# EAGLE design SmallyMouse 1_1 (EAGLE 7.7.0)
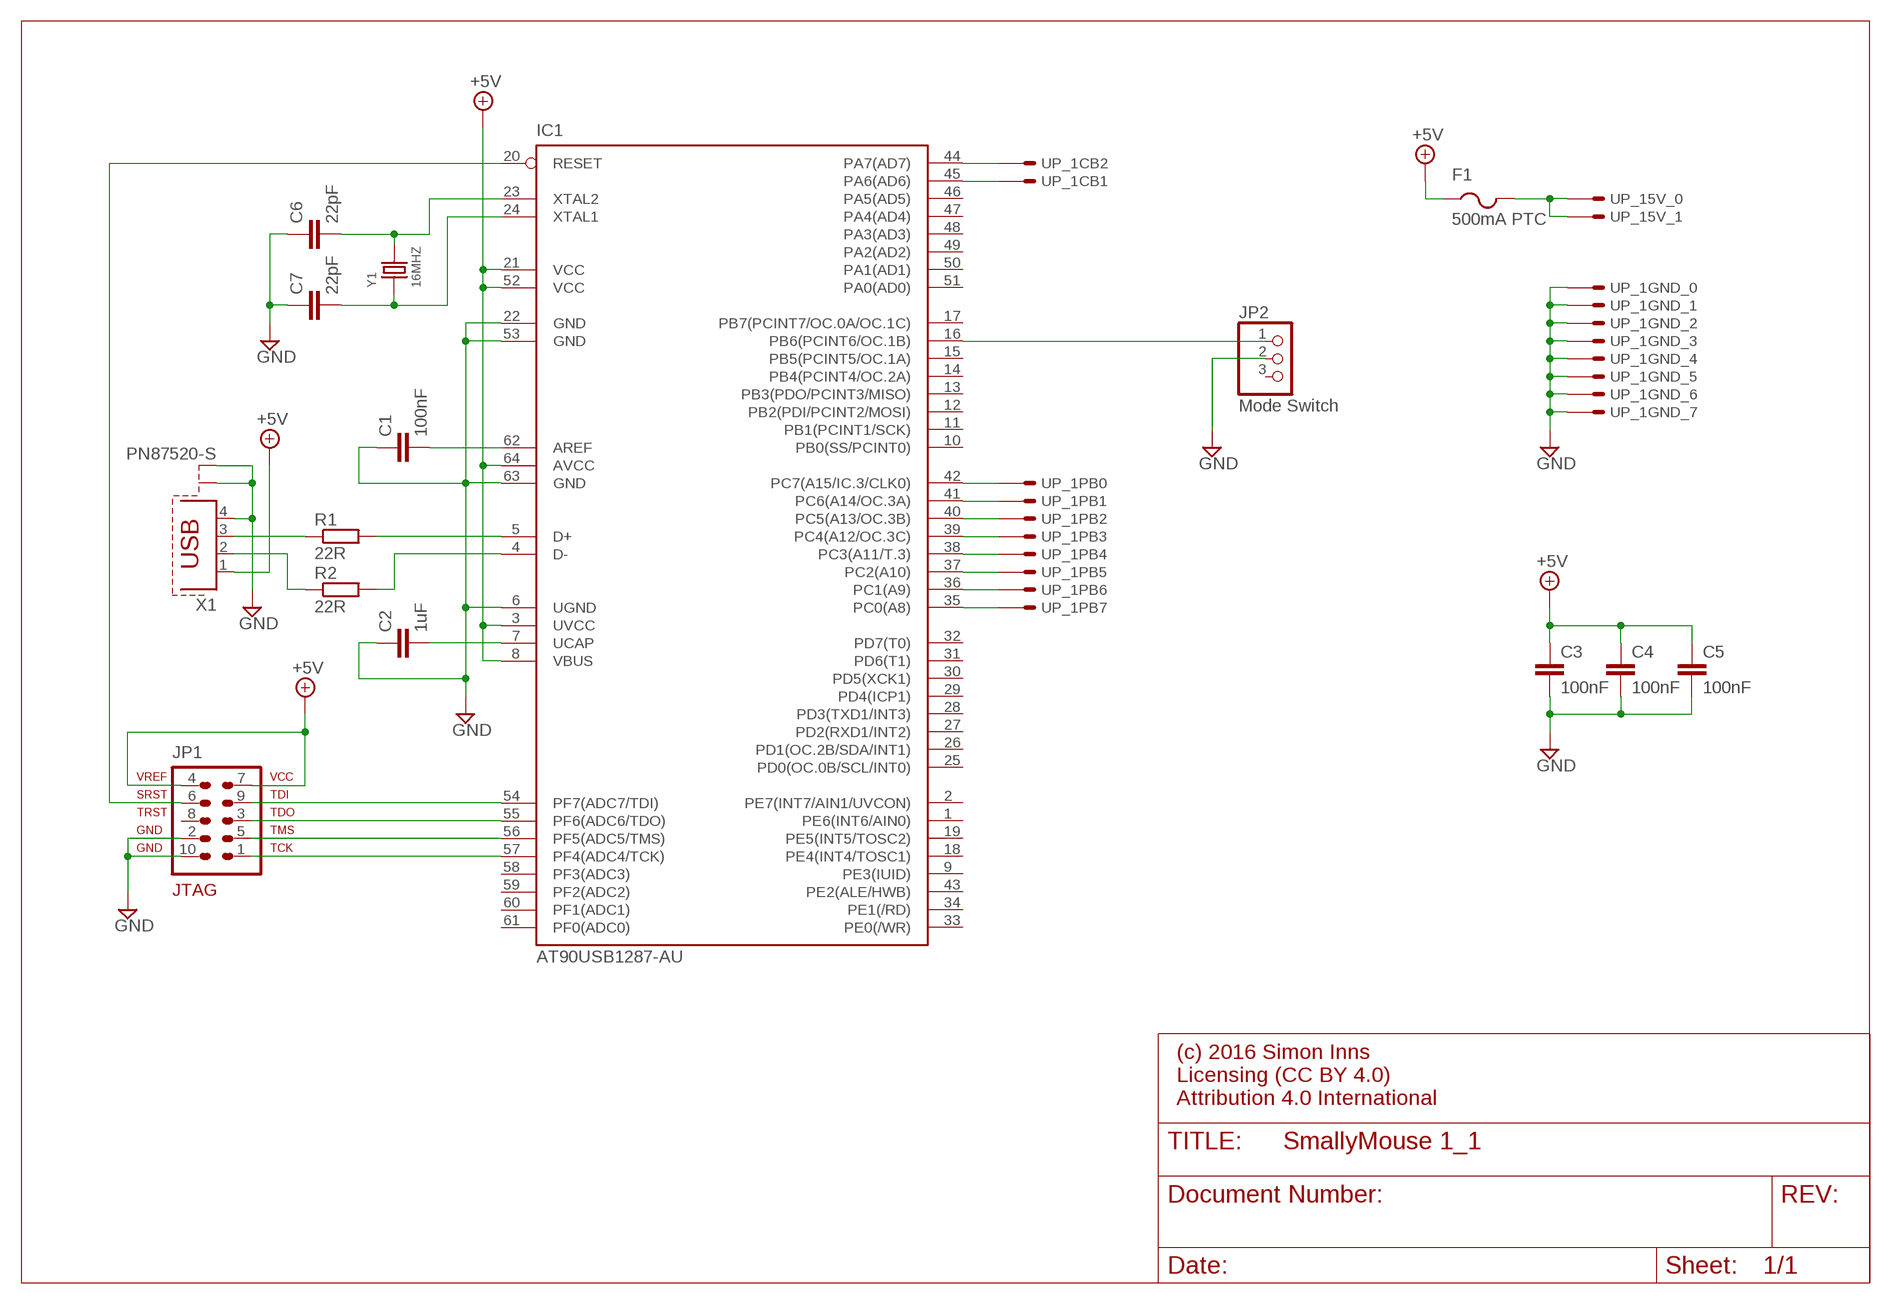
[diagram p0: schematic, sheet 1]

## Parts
C1  100nF  C-EUC0805  [C0805]
C2  1uF  C-EUC0805  [C0805]
C3  100nF  C-EUC0805  [C0805]
C4  100nF  C-EUC0805  [C0805]
C5  100nF  C-EUC0805  [C0805]
C6  22pF  C-EUC0805  [C0805]
C7  22pF  C-EUC0805  [C0805]
F1  500mA PTC  PTCFUSE-1812  [1812]
IC1  AT90USB1287-AU  [TQFP64]
JP1  AVR-JTAG-10  [AVR-JTAG-10]
JP2  Mode Switch  PINHD-1X3/90  [1X03/90]
R1  22R  R-EU_M1206  [M1206]
R2  22R  R-EU_M1206  [M1206]
UP_1  BBC_USERPORT  [20_PIN_HEADER]
X1  PN87520-S  [PN87520-S]
Y1  16MHZ  SMD-CRYSTAL-16MHZ-8PF-20PPM-40R(2P-5.0X3.2MM)  [X2-SMD-5.0X3.2X1.3MM]

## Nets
+5V: C3.1 C4.1 C5.1 F1.1 IC1.3(UVCC) IC1.8(VBUS) IC1.21(VCC) IC1.52(VCC) IC1.64(AVCC) JP1.4 JP1.7 X1.1
GND: C1.1 C2.1 C3.2 C4.2 C5.2 C6.1 C7.1 IC1.6(UGND) IC1.22(GND) IC1.53(GND) IC1.63(GND) JP1.2 JP1.10 JP2.2 UP_1.5 UP_1.7 UP_1.9 UP_1.11 UP_1.13 UP_1.15 UP_1.17 UP_1.19 X1.4 X1.S1 X1.S2
N$1: IC1.42(PC7(A15/IC.3/CLK0)) UP_1.6
N$2: IC1.41(PC6(A14/OC.3A)) UP_1.8
N$3: IC1.40(PC5(A13/OC.3B)) UP_1.10
N$4: IC1.39(PC4(A12/OC.3C)) UP_1.12
N$5: IC1.38(PC3(A11/T.3)) UP_1.14
N$6: IC1.37(PC2(A10)) UP_1.16
N$7: IC1.36(PC1(A9)) UP_1.18
N$8: IC1.35(PC0(A8)) UP_1.20
N$9: IC1.44(PA7(AD7)) UP_1.4
N$10: IC1.45(PA6(AD6)) UP_1.2
N$11: IC1.54(PF7(ADC7/TDI)) JP1.9
N$12: IC1.55(PF6(ADC6/TDO)) JP1.3
N$13: IC1.56(PF5(ADC5/TMS)) JP1.5
N$14: IC1.57(PF4(ADC4/TCK)) JP1.1
N$15: IC1.5(D+) R1.2
N$16: IC1.4(D-) R2.2
N$17: IC1.20(RESET) JP1.6
N$18: IC1.16(PB6(PCINT6/OC.1B)) JP2.1
N$19: F1.2 UP_1.1 UP_1.3
N$26: R1.1 X1.3
N$27: R2.1 X1.2
N$29: C1.2 IC1.62(AREF)
N$31: C2.2 IC1.7(UCAP)
N$32: C6.2 IC1.23(XTAL2) Y1.2
N$33: C7.2 IC1.24(XTAL1) Y1.1
Unconnected: IC1.1(PE6(INT6/AIN0)) IC1.2(PE7(INT7/AIN1/UVCON)) IC1.9(PE3(IUID)) IC1.10(PB0(SS/PCINT0)) IC1.11(PB1(PCINT1/SCK)) IC1.12(PB2(PDI/PCINT2/MOSI)) IC1.13(PB3(PDO/PCINT3/MISO)) IC1.14(PB4(PCINT4/OC.2A)) IC1.15(PB5(PCINT5/OC.1A)) IC1.17(PB7(PCINT7/OC.0A/OC.1C)) IC1.18(PE4(INT4/TOSC1)) IC1.19(PE5(INT5/TOSC2)) IC1.25(PD0(OC.0B/SCL/INT0)) IC1.26(PD1(OC.2B/SDA/INT1)) IC1.27(PD2(RXD1/INT2)) IC1.28(PD3(TXD1/INT3)) IC1.29(PD4(ICP1)) IC1.30(PD5(XCK1)) IC1.31(PD6(T1)) IC1.32(PD7(T0)) IC1.33(PE0(/WR)) IC1.34(PE1(/RD)) IC1.43(PE2(ALE/HWB)) IC1.46(PA5(AD5)) IC1.47(PA4(AD4)) IC1.48(PA3(AD3)) IC1.49(PA2(AD2)) IC1.50(PA1(AD1)) IC1.51(PA0(AD0)) IC1.58(PF3(ADC3)) IC1.59(PF2(ADC2)) IC1.60(PF1(ADC1)) IC1.61(PF0(ADC0)) JP1.8 JP2.3

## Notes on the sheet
- (c) 2016 Simon Inns
  Licensing (CC BY 4.0)
  Attribution 4.0 International

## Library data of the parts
C1-C7 = rcl:C-EU: CAPACITOR, European symbol
F1 = adafruit:PTCFUSE: PTC fuses, resettable thermistors
IC1 = at90usb:AT90USB1287-*: Atmel AT90USB1287 AVR Microcontroller with USB Interface and 128kB Flash Memory
JP1 = avr-7:AVR-JTAG-10: AVR JTAG Debug/Programming Header
JP2 = pinhead:PINHD-1X3: PIN HEADER
R1 R2 = rcl:R-EU_: RESISTOR, European symbol
UP_1 = BBC Micro:BBC_USERPORT: BBC Micro user port
X1 = con-berg:PN87520-S; OC_FARNELL: unknown; OC_NEWARK: unknown
Y1 = Seeed-OPL-Crystal-Oscillator:SMD-CRYSTAL-16MHZ-8PF-20PPM-40R(2P-5.0X3.2MM): 306010054; MPN: X053201602002

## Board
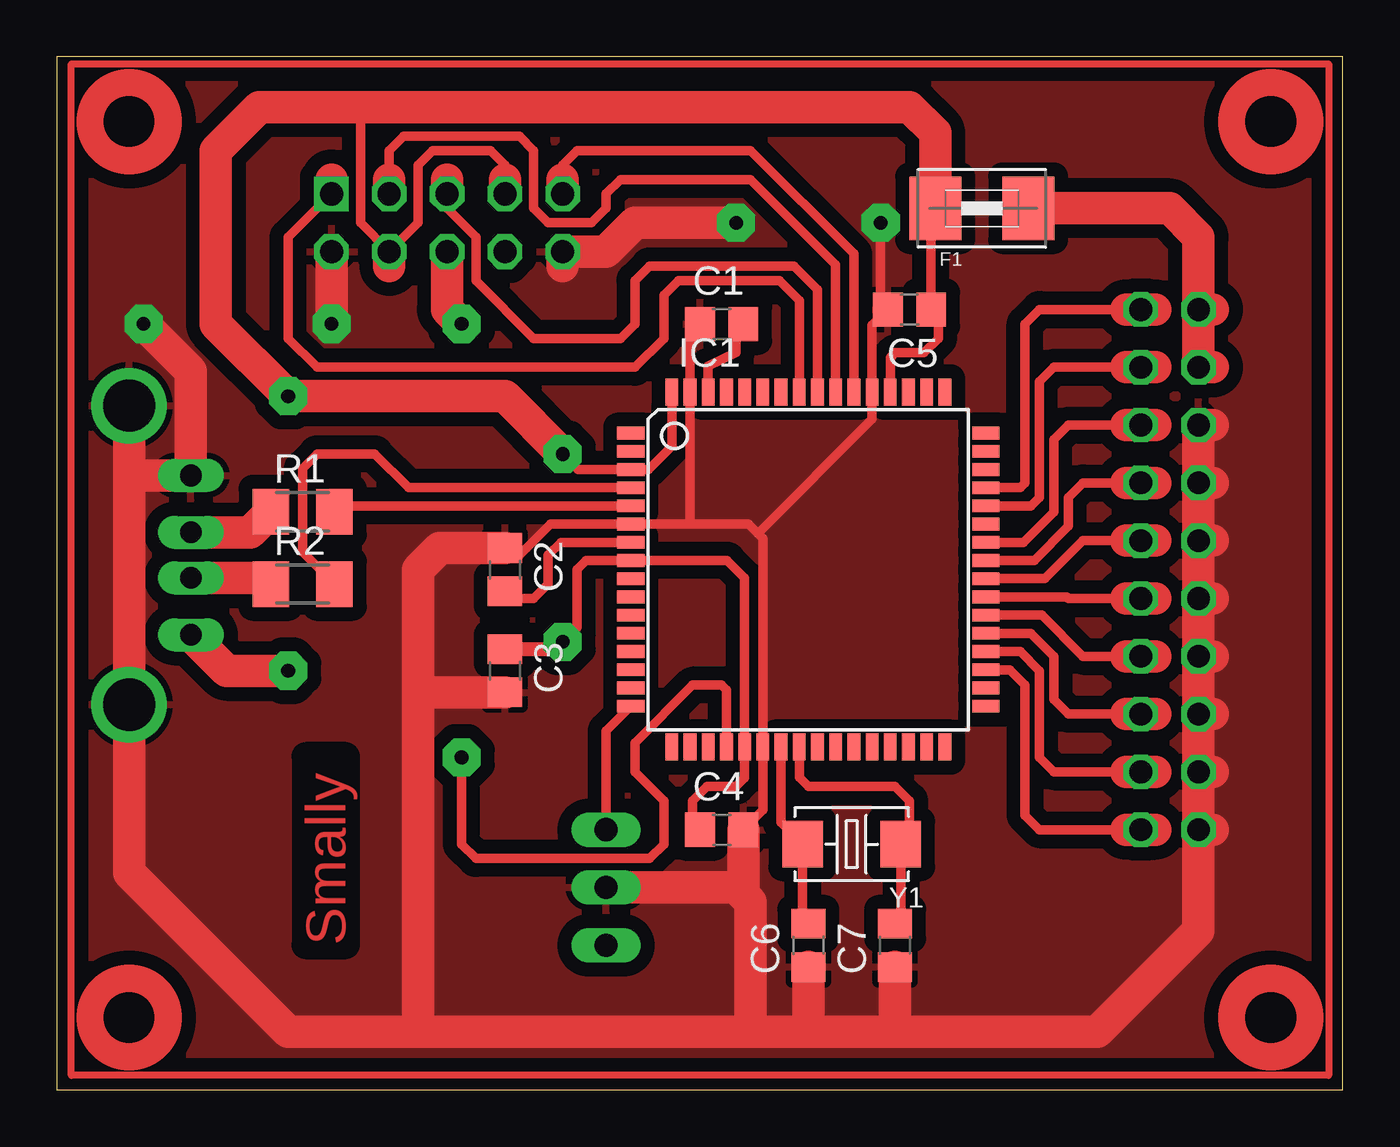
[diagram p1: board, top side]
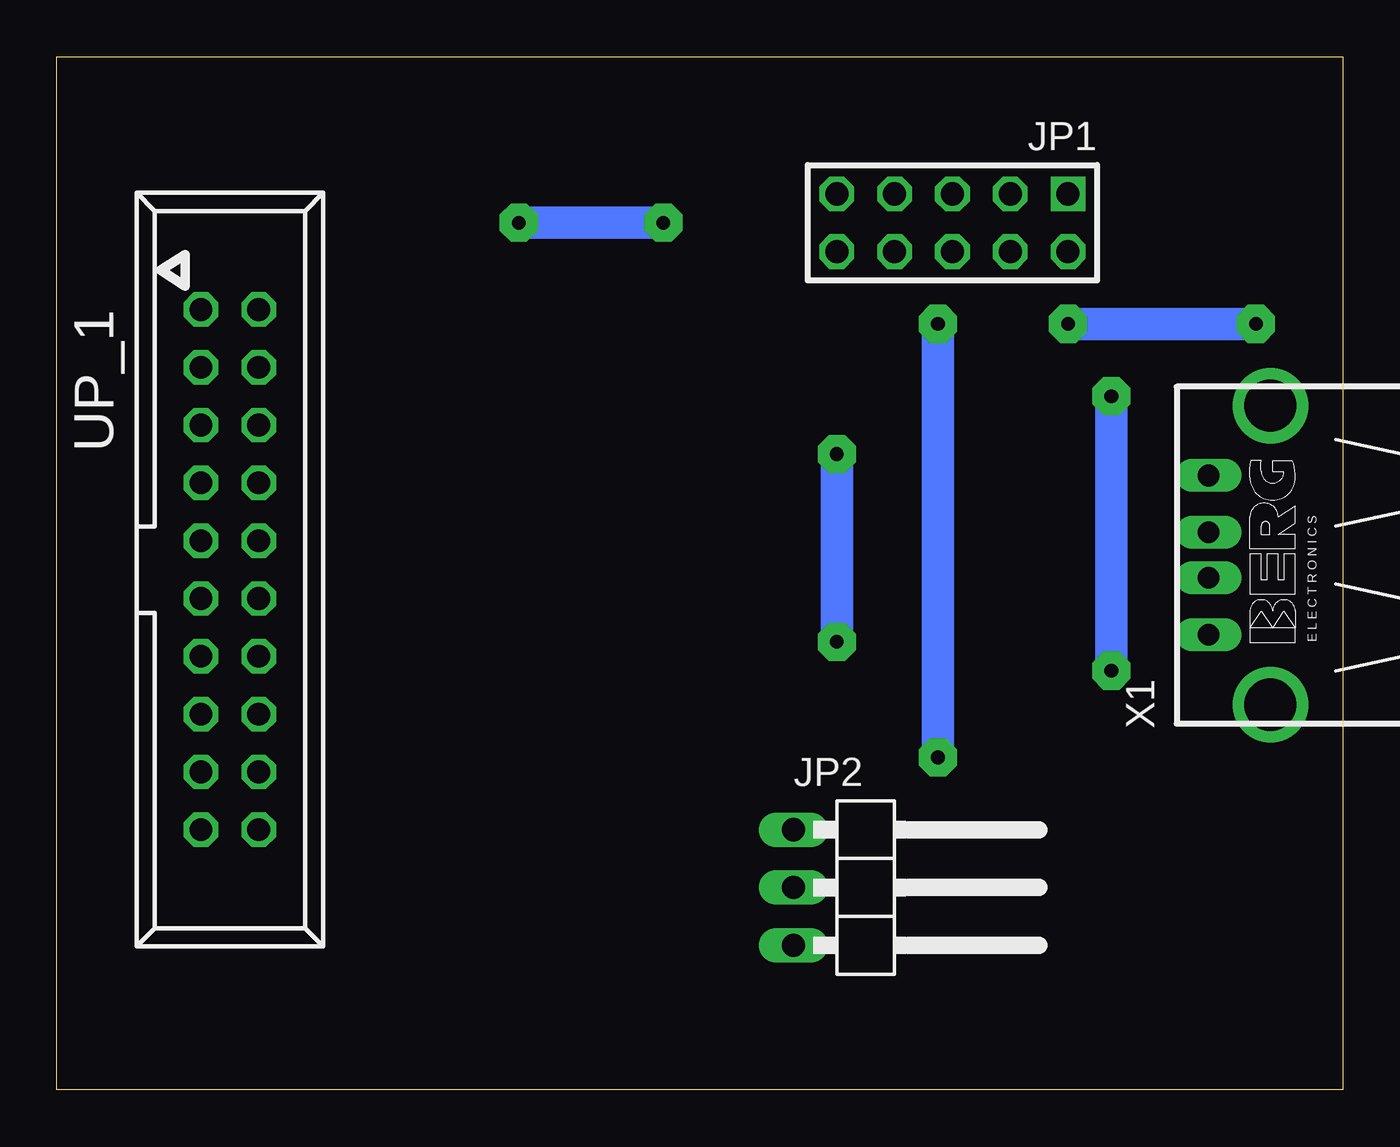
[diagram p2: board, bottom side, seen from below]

Size 56.49 x 45.39 mm. Coordinates in mm from the lower left corner, seen from the top.
Outline: 0,0 56.49,0 56.49,45.39 0,45.39 0,0
Copper layers (1*16): Top 0.035mm / dielectric 1.5mm / Bottom 0.035mm
Design rules "default": minimum track width 10mil, minimum drill 24mil, track to track 8mil, track to pad 8mil, pad to pad 8mil, via to via 8mil, smd to smd 8mil, copper to edge 40mil, drill to drill 8mil, minimum pad ring 10mil, minimum via ring 8mil, stop-mask expansion 4mil, vias tented up to drill 0mil, thermal gap 10mil
tRestrict: area 2.3,41.6 to 4.1,43.4; area 2.3,2.3 to 4.1,4.1; area 52.4,2.3 to 54.2,4.1; area 52.4,41.6 to 54.2,43.4

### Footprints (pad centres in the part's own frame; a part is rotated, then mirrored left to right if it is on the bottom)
C0805 = smd 1.3 x 1.5: 1 -0.95,0; 2 0.95,0
1812 = smd 2.286 x 2.794: 1 -2.046,0; 2 2.046,0
TQFP64 = smd 1.194 x 0.559: 1 -7.8,6; 2 -7.8,5.2; 3 -7.8,4.4; 4 -7.8,3.6; 5 -7.8,2.8; 6 -7.8,2; 7 -7.8,1.2; 8 -7.8,0.4; 9 -7.8,-0.4; 10 -7.8,-1.2; 11 -7.8,-2; 12 -7.8,-2.8; 13 -7.8,-3.6; 14 -7.8,-4.4; 15 -7.8,-5.2; 16 -7.8,-6; 33 7.8,-6; 34 7.8,-5.2; 35 7.8,-4.4; 36 7.8,-3.6; 37 7.8,-2.8; 38 7.8,-2; 39 7.8,-1.2; 40 7.8,-0.4; 41 7.8,0.4; 42 7.8,1.2; 43 7.8,2; 44 7.8,2.8; 45 7.8,3.6; 46 7.8,4.4; 47 7.8,5.2; 48 7.8,6 | smd 0.559 x 1.194: 17 -6,-7.8; 18 -5.2,-7.8; 19 -4.4,-7.8; 20 -3.6,-7.8; 21 -2.8,-7.8; 22 -2,-7.8; 23 -1.2,-7.8; 24 -0.4,-7.8; 25 0.4,-7.8; 26 1.2,-7.8; 27 2,-7.8; 28 2.8,-7.8; 29 3.6,-7.8; 30 4.4,-7.8; 31 5.2,-7.8; 32 6,-7.8; 49 6,7.8; 50 5.2,7.8; 51 4.4,7.8; 52 3.6,7.8; 53 2.8,7.8; 54 2,7.8; 55 1.2,7.8; 56 0.4,7.8; 57 -0.4,7.8; 58 -1.2,7.8; 59 -2,7.8; 60 -2.8,7.8; 61 -3.6,7.8; 62 -4.4,7.8; 63 -5.2,7.8; 64 -6,7.8
AVR-JTAG-10 = drill 1.016 square: 1 -5.08,-1.27 | drill 1.016 octagon: 2 -5.08,1.27; 3 -2.54,-1.27; 4 -2.54,1.27; 5 0,-1.27; 6 0,1.27; 7 2.54,-1.27; 8 2.54,1.27; 9 5.08,-1.27; 10 5.08,1.27
1X03/90 = drill 1.016 long: 1 -2.54,-3.81; 2 0,-3.81; 3 2.54,-3.81
M1206 = smd 1.6 x 2: 1 -1.4,0; 2 1.4,0
20_PIN_HEADER = drill 1 octagon: 1 -11.43,-1.27; 2 -11.43,1.27; 3 -8.89,-1.27; 4 -8.89,1.27; 5 -6.35,-1.27; 6 -6.35,1.27; 7 -3.81,-1.27; 8 -3.81,1.27; 9 -1.27,-1.27; 10 -1.27,1.27; 11 1.27,-1.27; 12 1.27,1.27; 13 3.81,-1.27; 14 3.81,1.27; 15 6.35,-1.27; 16 6.35,1.27; 17 8.89,-1.27; 18 8.89,1.27; 19 11.43,-1.27; 20 11.43,1.27
PN87520-S = drill 0.95 long: 1 -3.5,2.71; 2 -1,2.71; 3 1,2.71; 4 3.5,2.71 | drill 2.3 pad 2.9: S1 -6.57,0; S2 6.57,0
X2-SMD-5.0X3.2X1.3MM = smd 1.778 x 2.032: 1 -2.159,0; 2 2.159,0

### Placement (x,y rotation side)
C1  29.21,33.66 0 top
C2  19.68,22.86 270 top
C3  19.68,18.41 270 top
C4  29.21,11.43 0 top
C5  37.47,34.29 180 top
C6  33.02,6.35 90 top
C7  36.83,6.35 90 top
F1  40.64,38.73 0 top
IC1  33.02,22.86 0 top
JP1  17.14,38.1 180 bottom
JP2  20.32,8.89 270 bottom
R1  10.79,25.4 0 top
R2  10.79,22.23 0 top
UP_1  48.9,22.86 270 bottom
X1  3.17,23.5 90 bottom
Y1  34.92,10.79 180 top

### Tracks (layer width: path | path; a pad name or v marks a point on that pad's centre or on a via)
+5V  (via drill 0.6 pad 1.68)
  Top 0.406: C4.1 27.94,11.75 27.94,12.7 28.57,13.34 29.84,13.34 30.22,13.71 IC1.21 30.22,22.48 29.45,23.26 IC1.8 23.26,23.26 22.86,22.86 22.86,20.32 v22.23,19.68 | IC1.52 36.62,32.17 36.83,32.38 38.1,32.38 38.73,33.02 38.73,33.97 C5.1 38.41,38.56 F1.1 | IC1.64 27.02,28.29 25.99,27.26 IC1.3 22.91,27.26 v22.23,27.94 | 19.68,40.01 19.68,40.64 19.05,41.27 16.51,41.27 15.88,40.64 15.88,38.1 JP1.4 13.34,38.1 13.34,43.18
  Top 0.61: C3.1 21.91,19.36 v22.23,19.68
  Top 1.422: F1.1 38.59,42.05 37.47,43.18 13.34,43.18 8.89,43.18 6.99,41.27 6.99,33.66 v10.16,30.48 19.68,30.48 v22.23,27.94 | X1.1 7.46,18.41 v10.16,18.41 | JP1.7 19.68,40.01 | JP1.4 14.61,36.2
  Bottom 1.422: v10.16,18.41 v10.16,30.48 | v22.23,19.68 v22.23,27.94
GND  (via drill 0.6 pad 1.68)
  Top 0.406: C4.2 31.02,12.29 IC1.22 31.02,24.23 30.8,24.45 | C1.1 27.82,33.85 IC1.63 27.82,24.98 27.94,24.86 | 30.8,24.45 30.39,24.86 27.94,24.86 | 27.94,24.86 IC1.6 21.68,24.86 20.32,23.5 19.68,24.13 | 30.8,24.45 35.82,29.47 IC1.53 35.82,33.59 C5.2 36.2,34.61 v36.2,38.1
  Top 1.422: UP_1.19 UP_1.17 | UP_1.17 UP_1.15 | UP_1.15 UP_1.13 | UP_1.13 UP_1.11 | UP_1.11 UP_1.9 | UP_1.9 UP_1.7 | UP_1.7 UP_1.5 50.8,29.21 | 33.02,2.54 36.83,2.54 | 36.83,2.54 45.72,2.54 50.16,6.99 UP_1.19 | JP2.2 29.84,8.89 30.16,8.57 | 15.88,2.54 10.16,2.54 3.17,9.53 X1.S1 3.17,27 | 15.88,2.54 30.48,2.54 | 30.48,2.54 33.02,2.54 | 3.17,27 X1.S2 | 3.17,27 X1.4 5.88,31.58 v3.81,33.66 | C2.1 16.82,23.81 15.88,22.86 15.88,17.14 | 15.88,17.14 15.88,2.54 | C3.2 16.2,17.46 15.88,17.14 | C7.1 36.83,2.54 | C6.1 33.02,2.54 | 30.48,2.54 30.48,8.26 30.16,8.57 | C4.2 30.16,8.57 | JP1.2 v12.06,33.66 | v29.84,38.1 25.4,38.1 24.13,36.83 JP1.10 22.23,36.2 | UP_1.19 50.8,11.43 | UP_1.17 50.8,13.97 | UP_1.15 50.8,16.51 | UP_1.13 50.8,19.05 | UP_1.11 50.8,21.59 | UP_1.9 50.8,24.13 | UP_1.7 50.8,26.67
  Bottom 1.422: v12.06,33.66 v3.81,33.66 | v29.84,38.1 v36.2,38.1
  pour Top (isolate 0.61): 0,45.09 56.52,45.09 56.52,0.64 0,0.64
N$1
  Top 0.406: IC1.42 42.48,24.06 43.81,25.4 43.81,28.57 44.45,29.21 46.99,29.21
  Top 1.422: 46.99,29.21 UP_1.6 48.26,29.21
N$2
  Top 0.406: IC1.41 42.95,23.26 44.45,24.77 44.45,26.04 45.09,26.67 46.99,26.67
  Top 1.422: 46.99,26.67 UP_1.8 48.26,26.67
N$3
  Top 0.406: IC1.40 43.41,22.46 45.09,24.13 46.99,24.13
  Top 1.422: 46.99,24.13 UP_1.10 48.26,24.13
N$4
  Top 0.406: IC1.39 44.38,21.66 44.45,21.59 46.99,21.59
  Top 1.422: 46.99,21.59 UP_1.12 48.26,21.59
N$5
  Top 0.406: IC1.38 43.27,20.86 45.09,19.05 46.99,19.05
  Top 1.422: 46.99,19.05 UP_1.14 48.26,19.05
N$6
  Top 0.406: IC1.37 42.8,20.06 43.81,19.05 43.81,17.14 44.45,16.51 46.99,16.51
  Top 1.422: 46.99,16.51 UP_1.16 48.26,16.51
N$7
  Top 0.406: IC1.36 42.34,19.26 43.18,18.41 43.18,14.61 43.81,13.97 46.99,13.97
  Top 1.422: 46.99,13.97 UP_1.18 48.26,13.97
N$8
  Top 0.406: IC1.35 41.87,18.46 42.55,17.78 42.55,12.06 43.18,11.43 46.99,11.43
  Top 1.422: 46.99,11.43 UP_1.20 48.26,11.43
N$9
  Top 0.406: IC1.44 42.8,25.66 43.18,26.04 43.18,31.11 43.81,31.75 46.99,31.75
  Top 1.422: 46.99,31.75 UP_1.4 48.26,31.75
N$10
  Top 0.406: IC1.45 42.34,26.46 42.55,26.67 42.55,33.66 43.18,34.29 46.99,34.29
  Top 1.422: 46.99,34.29 UP_1.2 48.26,34.29
N$11
  Top 0.406: 22.23,40.01 22.23,40.64 22.86,41.27 30.48,41.27 35.02,36.73 IC1.54
  Top 1.422: JP1.9 22.23,40.01
N$12
  Top 0.406: 14.61,40.01 14.61,41.27 15.24,41.91 20.32,41.91 20.95,41.27 20.95,38.73 21.59,38.1 23.5,38.1 24.13,38.73 24.13,39.37 24.77,40.01 30.48,40.01 34.22,36.27 IC1.55
  Top 1.422: JP1.3 14.61,40.01
N$13
  Top 0.406: IC1.56 33.42,35.16 32.38,36.2 26.04,36.2 25.4,35.56 25.4,33.66 24.77,33.02 20.95,33.02 18.41,35.56 18.41,37.47 17.14,38.73 JP1.5
  Top 1.422: JP1.5 17.14,40.01
N$14
  Top 0.406: IC1.57 32.62,34.69 31.75,35.56 27.3,35.56 26.67,34.92 26.67,33.02 25.4,31.75 11.43,31.75 10.16,33.02 10.16,37.47 JP1.1
  Top 1.422: JP1.1 12.06,40.01
N$15
  Top 0.406: IC1.5 12.57,25.66 R1.2
N$16
  Top 0.406: IC1.4 15.45,26.46 13.97,27.94 11.43,27.94 10.79,27.3 10.79,23.62 R2.2
N$17  (via drill 0.6 pad 1.68)
  Top 0.406: IC1.20 29.42,17.57 29.21,17.78 27.94,17.78 25.4,15.24 25.4,13.97 26.67,12.7 26.67,10.79 26.04,10.16 18.41,10.16 17.78,10.79 v17.78,14.61
  Top 1.422: JP1.6 17.14,34.29 v17.78,33.66
  Bottom 1.422: v17.78,14.61 v17.78,33.66
N$18
  Top 0.406: IC1.16 24.13,15.77 JP2.1
N$19
  Top 1.422: UP_1.1 UP_1.3 50.8,31.75 | UP_1.1 50.16,37.47 48.9,38.73 F1.2 | UP_1.1 50.8,34.29
N$20
  pour Top (isolate 0.61): 0,45.09 55.88,45.09 55.88,0.64 0,0.64
N$21
  Top 0.305: 0.64,45.09 55.88,45.09 55.88,0.64 0.64,0.64 0.64,45.09
N$26
  Top 1.422: X1.3 8.49,24.5 R1.1
N$27
  Top 1.422: X1.2 9.12,22.5 R2.1
N$29
  Top 0.406: IC1.62 28.62,31.8 29.84,32.38 29.84,33.98 C1.2
N$31
  Top 0.406: IC1.7 22.16,24.06 21.59,23.5 21.59,22.23 20.95,21.59 20,21.59 C2.2
N$32
  Top 0.406: IC1.23 31.82,11.74 Y1.2 32.77,7.55 C6.2
N$33
  Top 0.406: IC1.24 32.62,13.73 33.02,13.34 36.83,13.34 37.47,12.7 37.47,11.18 Y1.1 37.08,7.55 C7.2
(copper drawn outside any net)
  shapes: Top circle x8

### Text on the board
Top: Smally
